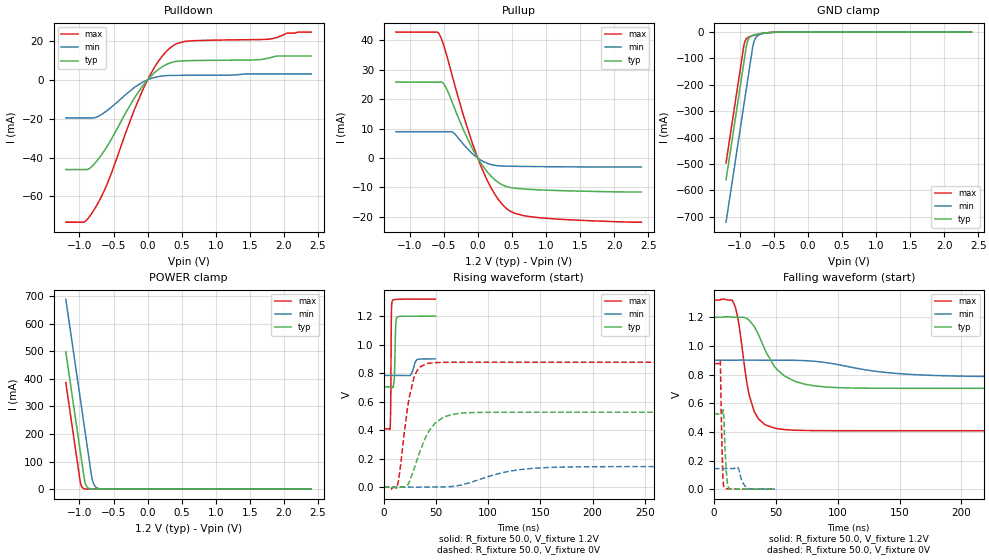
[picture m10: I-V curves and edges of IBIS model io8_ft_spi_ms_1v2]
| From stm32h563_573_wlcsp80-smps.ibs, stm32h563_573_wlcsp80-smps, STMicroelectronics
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[Model]   io8_ft_spi_ms_1v2
Model_type I/O
Polarity   Non-Inverting
Enable   Active-Low
| CAP_THRESHOLD on pad IOFT is "UDTCAPC" :
| Rising=20.0% of vddiom   Falling=80.0% of vddiom
| C_comp min and max val. don't necessarily correlate with the min and max pvt
| but are the smallest and greatest pad capacitance found.
| var   typ   min   max
C_comp   4.02960pF  3.92715pF  4.03450pF
|C_comp_pullup   2.45865pF  2.27005pF  2.18290pF
|C_comp_pulldown   1.57095pF  1.65710pF  1.85160pF
Vinl = 270.0mV
Vinh = 924.0mV
Vmeas = 600.0mV   | Reference voltage for timing measurements
Cref  = 50.0pF   | Timing specification test load capacitance value
Rref  = 100.0MOhm   | Timing specification test load resistance value
Vref  = 600.0mV   | Timing specification test load voltage
[Model Spec]
| TIME_THRESHOLD on pin ZIV11 is "CMOS" :
| Rising=40.0% of vdd   Falling=60.0% of vdd
Vinl 447.80000mV 344.80000mV 489.80000mV
Vinh 733.20000mV 535.20000mV 813.20000mV
| variable   typ   min   max
[Temperature Range] 25.0 125.0 -40.0
| variable   typ   min   max
[Voltage Range] 1.2V 900.0mV 1.32V
| variable   typ   min   max
[POWER Clamp Reference] 1.2V 900.0mV 1.32V
| variable   typ   min   max
[GND Clamp Reference] 0V 0V 0V
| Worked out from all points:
|   slope of the pulldown table from 0 to 0.18 V, typ, clamps not added: 30.6 ohm
|   slope of the pullup table from 0 to 0.18 V, typ, clamps not added: 31.3 ohm
|   GND clamp passes 1 mA (typ) near -0.52 V on its own axis
|   POWER clamp passes 1 mA (typ) near -0.84 V on its own axis
|   rising waveform, R_fixture 50.0, V_fixture 1.2V: 20-80 % time 1.03ns typ, 2.95ns min, 541ps max; typ from 0.704 V to 1.2 V
|   falling waveform, R_fixture 50.0, V_fixture 1.2V: 20-80 % time 20.6ns typ, 53.7ns min, 10.4ns max; typ from 1.2 V to 0.704 V
|   rising waveform, R_fixture 50.0, V_fixture 0V: 20-80 % time 18.1ns typ, 42.4ns min, 10.3ns max; typ from 0 V to 0.525 V
|   falling waveform, R_fixture 50.0, V_fixture 0V: 20-80 % time 1.84ns typ, 3.78ns min, 1.35ns max; typ from 0.525 V to 0 V
[POWER Clamp]
-1.2V     497.8mA    689.2mA    386.5mA
-990mV    140.8mA    332.2mA    29.53mA
-980mV    123.8mA    315.2mA    17.95mA
-960mV    89.81mA    281.2mA    6.634mA
-930mV    38.81mA    230.2mA    1.49mA
-900mV    12.07mA    179.2mA    334.8uA
-870mV    3.756mA    128.2mA    75.22uA
-820mV    536.4uA    44.98mA    6.246uA
-790mV    166.9uA    18.76mA    1.403uA
-750mV    35.18uA    5.846mA    191.9nA
-590mV    70.48nA    54.99uA    204.6pA
2.4V      0A         0A         0A
[GND Clamp]
-1.2V     -559.6mA   -720.6mA   -495.5mA
-940mV    -117.6mA   -278.6mA   -53.46mA
-930mV    -100.6mA   -261.6mA   -41.27mA
-900mV    -50.49mA   -210.6mA   -24.86mA
-880mV    -31.4mA    -176.6mA   -20.57mA
-850mV    -18.9mA    -125.6mA   -16.88mA
-810mV    -12.57mA   -58.3mA    -13.49mA
-780mV    -10.11mA   -29.57mA   -11.38mA
-740mV    -7.754mA   -14.31mA   -8.91mA
-640mV    -3.713mA   -4.821mA   -4.078mA
-390mV    -82.2uA    -288.6uA   -29.73uA
2.4V      3.859nA    727.3nA    172.3pA
| variable   typ   min   max
[Pullup Reference] 1.2V 900.0mV 1.32V
| variable   typ   min   max
[Pulldown Reference] 0V 0V 0V
[Pullup]
-1.2V     25.83mA    8.95mA     42.8mA
-570mV    25.83mA    8.95mA     42.28mA
-490mV    24.91mA    8.95mA     37.64mA
-360mV    18.1mA     8.66mA     26.77mA
-200mV    9.064mA    4.389mA    13.74mA
0V        7.46pA     726pA      4.231pA
220mV     -6.707mA   -2.341mA   -11.11mA
330mV     -8.708mA   -2.669mA   -14.91mA
440mV     -9.808mA   -2.753mA   -17.46mA
670mV     -10.5mA    -2.846mA   -19.55mA
900mV     -10.8mA    -2.907mA   -20.25mA
2.4V      -11.52mA   -3.045mA   -21.79mA
[Pulldown]
-1.2V     -46.17mA   -19.62mA   -73.27mA
-930mV    -46.17mA   -19.62mA   -73.17mA
-770mV    -42.8mA    -19.41mA   -66.04mA
-570mV    -32.88mA   -15.18mA   -51.58mA
-200mV    -9.658mA   -4.083mA   -15.89mA
-80mV     -3.488mA   -1.363mA   -5.887mA
130mV     4.529mA    1.468mA    8.049mA
340mV     8.782mA    2.251mA    16.66mA
540mV     9.805mA    2.305mA    19.74mA
1.79V     11.29mA    3.028mA    20.92mA
2.05V     12.25mA    3.028mA    24.04mA
2.4V      12.25mA    3.028mA    24.55mA
[Ramp]
dV/dt_r 315.14646mV/17.68534ns 86.07509mV/42.12255ns 525.78086mV/9.87734ns
dV/dt_f 297.79755mV/20.21461ns 69.90491mV/53.29231ns 547.13927mV/10.11944ns
R_load = 50.0
| Removed startup time: 0s 0s 0s  .
| Removed end time: 49.4ns.
[Rising Waveform]
R_fixture   = 50.0
V_fixture   = 1.2V
V_fixture_min = 900.0mV
V_fixture_max = 1.32V
0s        703.7mV    783.5mV    408.1mV
6.25ns    703.7mV    783.5mV    420.4mV
6.75ns    703.8mV    783.5mV    583.4mV
7.4ns     703.8mV    783.5mV    1.199V
8.05ns    702.4mV    783.5mV    1.303V
10.1ns    753.2mV    783.5mV    1.316V
11.65ns   1.147V     783.5mV    1.317V
13.1ns    1.195V     783.5mV    1.318V
32.3ns    1.2V       895.9mV    1.32V
49.4ns    1.2V       899.7mV    1.32V
| Removed startup time: 0s 0s 0s  .
| Removed end time: 399.4ns.
[Falling Waveform]
R_fixture   = 50.0
V_fixture   = 1.2V
V_fixture_min = 900.0mV
V_fixture_max = 1.32V
0s        1.2V       900mV      1.32V
16.3ns    1.2V       899.9mV    1.295V
20.2ns    1.2V       900.9mV    1.154V
27.75ns   1.185V     900.8mV    692.3mV
32.6ns    1.137V     900.8mV    542.6mV
48.9ns    858mV      900mV      426.9mV
65.2ns    753.6mV    899.6mV    411.7mV
97.8ns    709.7mV    873.6mV    408.2mV
179.4ns   703.7mV    793.3mV    408.1mV
399.4ns   703.7mV    783.5mV    408.1mV
| Removed startup time: 0s 0s 0s  .
| Removed end time: 399.4ns.
[Rising Waveform]
R_fixture   = 50.0
V_fixture   = 0V
V_fixture_min = 0V
V_fixture_max = 0V
0s        166.5nV    850.9nV    114.4nV
13.3ns    -1.886mV   911.3nV    15.21mV
15.3ns    -471.3uV   555.4nV    100mV
24.5ns    34.33mV    -139.9uV   630mV
31.5ns    180.1mV    -2.029mV   810.9mV
40.4ns    352.9mV    -71.49uV   864mV
57.1ns    490.1mV    590.8uV    875.5mV
73.4ns    518.2mV    12.37mV    876.1mV
146.8ns   525.1mV    133mV      876.3mV
399.4ns   525.2mV    143.5mV    876.3mV
| Removed startup time: 0s 0s 0s  .
| Removed end time: 49.4ns.
[Falling Waveform]
R_fixture   = 50.0
V_fixture   = 0V
V_fixture_min = 0V
V_fixture_max = 0V
0s        525.3mV    143.6mV    876.3mV
5.25ns    525.3mV    143.6mV    890.9mV
6ns       524.7mV    143.6mV    532.8mV
7.05ns    534.9mV    143.6mV    169.3mV
8.15ns    501.9mV    143.6mV    15.75mV
10ns      137mV      143.6mV    3.693mV
12.1ns    7.135mV    143.6mV    2.298mV
19.15ns   737.6uV    154.9mV    863.6uV
27.25ns   539.2uV    7.611mV    231.6uV
49.4ns    117uV      87.85uV    21.78uV
